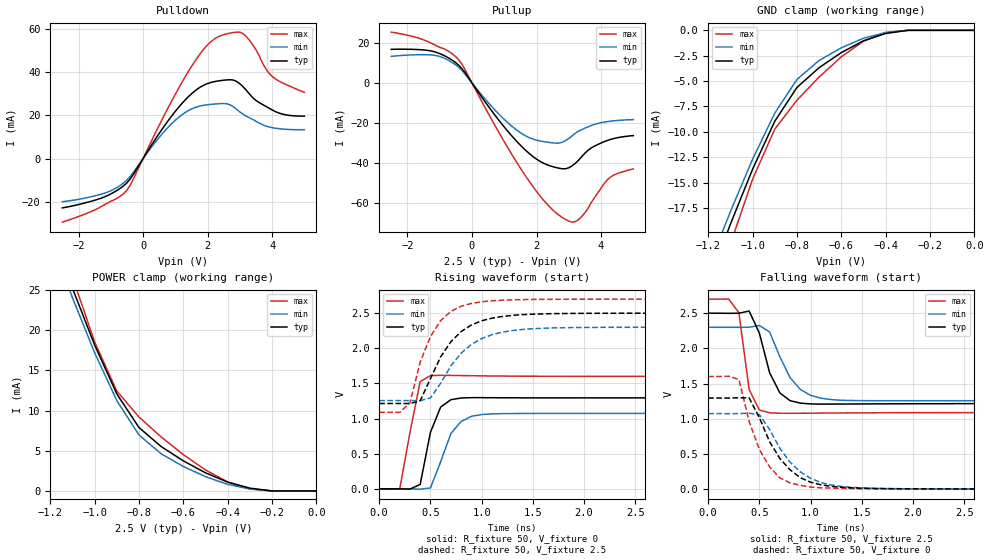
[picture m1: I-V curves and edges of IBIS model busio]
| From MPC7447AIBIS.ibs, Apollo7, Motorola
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| *   busio Model   *
[Model]   busio
Model_type   I/O
Polarity   Non-Inverting
Vinl = 0.5V
Vinh = 1.7V
Vmeas = 1.25V
Cref = 0
Rref = 50
Vref = 1.25V
|   typ   min   max
C_comp   3.929453e-12   3.101988e-12   4.107415e-12
|   typ   min   max
[Voltage range]   2.5V   2.3V   2.7V
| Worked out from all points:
|   slope of the pulldown table from 0 to 0.375 V, typ, clamps not added: 42.4 ohm
|   slope of the pullup table from 0 to 0.375 V, typ, clamps not added: 43.1 ohm
|   GND clamp passes 1 mA (typ) near -0.50 V on its own axis
|   POWER clamp passes 1 mA (typ) near -0.39 V on its own axis
|   falling waveform, R_fixture 50, V_fixture 2.5: 20-80 % time 172ps typ, 230ps min, 89.2ps max; typ from 2.5 V to 1.22 V
|   rising waveform, R_fixture 50, V_fixture 0: 20-80 % time 138ps typ, 188ps min, 126ps max; typ from 0 V to 1.29 V
|   falling waveform, R_fixture 50, V_fixture 0: 20-80 % time 321ps typ, 339ps min, 252ps max; typ from 1.29 V to 0 V
|   rising waveform, R_fixture 50, V_fixture 2.5: 20-80 % time 336ps typ, 362ps min, 261ps max; typ from 1.22 V to 2.5 V
[Pulldown]
|   Voltage   I(typ)   I(min)   I(max)
-2.5V     -22.81mA   -19.95mA   -29.44mA
-1.2V     -17.76mA   -16.03mA   -21.41mA
-500mV    -11.21mA   -9.919mA   -14.62mA
500mV     11.65mA    9.811mA    15.41mA
1.1V      23.71mA    19.06mA    32.51mA
1.8V      33.34mA    24.47mA    49.14mA
2.3V      35.89mA    25.37mA    56.19mA
2.8V      36.37mA    24mA       58.39mA
3.1V      33.29mA    20.57mA    57.86mA
3.5V      26.94mA    17.3mA     50.4mA
4V        22.56mA    14.35mA    38.1mA
5V        19.65mA    13.41mA    30.74mA
[GND_clamp]
-2.5V     -110.4mA   -105.1mA   -127.7mA
-1.2V     -24.9mA    -23.38mA   -27.95mA
-1.1V     -19.1mA    -17.86mA   -21.05mA
-1V       -13.68mA   -12.7mA    -14.67mA
-900mV    -8.957mA   -8.162mA   -9.74mA
-800mV    -5.626mA   -4.838mA   -6.885mA
-700mV    -3.677mA   -2.97mA    -4.599mA
-600mV    -2.195mA   -1.723mA   -2.612mA
-500mV    -1.034mA   -780.8uA   -1.071mA
-400mV    -309.9uA   -222.9uA   -209.9uA
-300mV    0A         0A         0A
0V        0A         0A         0A
[Pullup]
-2.5V     16.79mA    13.3mA     25.4mA
-1.1V     15.26mA    13.64mA    18.55mA
-400mV    8.678mA    7.673mA    11.35mA
700mV     -15.83mA   -13.3mA    -20.88mA
1.5V      -31.05mA   -24.82mA   -42.49mA
2.2V      -39.92mA   -29.22mA   -58.16mA
2.9V      -42.83mA   -28.75mA   -68.13mA
3.1V      -41.39mA   -26.43mA   -69.49mA
3.3V      -38.62mA   -24.09mA   -68.22mA
3.7V      -32.39mA   -21.2mA    -59.6mA
4.2V      -28.67mA   -19.26mA   -48.23mA
5V        -26.27mA   -18.29mA   -42.92mA
[POWER_clamp]
-2.5V     145.7mA    140mA      164.2mA
-1.1V     25.21mA    24.04mA    26.61mA
-1V       18.15mA    17.19mA    18.53mA
-900mV    12.07mA    11.24mA    12.42mA
-800mV    7.883mA    6.957mA    9.197mA
-700mV    5.518mA    4.618mA    6.718mA
-600mV    3.739mA    3.044mA    4.507mA
-500mV    2.251mA    1.774mA    2.605mA
-400mV    1.088mA    814.2uA    1.123mA
-300mV    343.1uA    240.3uA    250.5uA
-200mV    0A         0A         0A
0V        0A         0A         0A
|   typ   min   max
[Ramp]
dV/dt_r   0.77685/1.19698e-10   0.64397/1.67498e-10   0.96056/7.01159e-11
dV/dt_f   0.77079/1.56725e-10   0.62574/2.18710e-10   0.96651/8.83620e-11
[Falling Waveform]
R_fixture = 50
V_fixture = 2.5
V_fixture_min = 2.3
V_fixture_max = 2.7
| time   V(typ)   V(min)   V(max)
0s        2.5V       2.3V       2.7V
200ps     2.498V     2.3V       2.701V
300ps     2.5V       2.299V     2.506V
400ps     2.531V     2.301V     1.414V
500ps     2.217V     2.325V     1.125V
600ps     1.655V     2.234V     1.085V
700ps     1.367V     1.882V     1.079V
900ps     1.223V     1.417V     1.079V
1.3ns     1.209V     1.263V     1.083V
19.7ns    1.215V     1.257V     1.089V
[Rising Waveform]
R_fixture = 50
V_fixture = 0
V_fixture_min = 0
V_fixture_max = 0
| time   V(typ)   V(min)   V(max)
0s        228.6uV    237.9uV    194.3uV
200ps     848.3uV    -206.3uV   -2.886mV
400ps     63.85mV    -3.455mV   1.527V
500ps     804.3mV    14.31mV    1.611V
600ps     1.164V     385.6mV    1.616V
700ps     1.269V     787.8mV    1.614V
800ps     1.293V     959.2mV    1.612V
900ps     1.298V     1.032V     1.61V
1.1ns     1.297V     1.067V     1.606V
19.7ns    1.295V     1.074V     1.601V
[Falling Waveform]
R_fixture = 50
V_fixture = 0
V_fixture_min = 0
V_fixture_max = 0
| time   V(typ)   V(min)   V(max)
0s        1.295V     1.074V     1.601V
300ps     1.299V     1.074V     1.558V
400ps     1.297V     1.079V     961.9mV
500ps     1.016V     1.058V     565.4mV
600ps     673.6mV    846.9mV    315.8mV
700ps     436.8mV    580.7mV    160.7mV
900ps     163.5mV    246mV      54.49mV
1.1ns     62.11mV    94.9mV     19.72mV
2.2ns     3.93mV     4.082mV    2.872mV
19.7ns    242.4uV    257uV      198.4uV
[Rising Waveform]
R_fixture = 50
V_fixture = 2.5
V_fixture_min = 2.3
V_fixture_max = 2.7
| time   V(typ)   V(min)   V(max)
0s        1.215V     1.257V     1.089V
200ps     1.215V     1.257V     1.088V
300ps     1.214V     1.257V     1.224V
400ps     1.253V     1.255V     1.804V
500ps     1.568V     1.295V     2.166V
600ps     1.879V     1.502V     2.394V
800ps     2.238V     1.931V     2.598V
1.1ns     2.428V     2.193V     2.676V
2.2ns     2.498V     2.298V     2.698V
19.7ns    2.5V       2.3V       2.7V
